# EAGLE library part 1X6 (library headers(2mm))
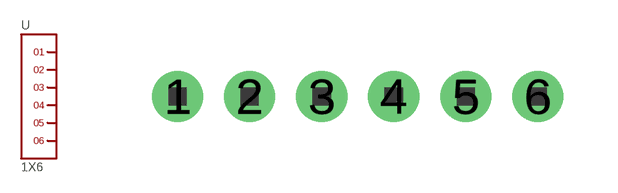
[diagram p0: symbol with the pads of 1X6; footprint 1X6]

Designator prefix -

## 1X6  [1X6]
1  1
2  2
3  3
4  4
5  5
6  6

## Footprint 1X6 (pad centres in mm)
drill 0.8 pad 1.422: 1 -5,0; 2 -3,0; 3 -1,0; 4 1,0; 5 3,0; 6 5,0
